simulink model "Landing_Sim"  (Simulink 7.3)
settings: Solver=ode45  StartTime=0.0  StopTime=80  RelTol=1e-3
InitFcn:
  | init
StopFcn:
  | pl
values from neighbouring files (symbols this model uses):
  calfa = cos(alfa0*d2r)    [init.m]
  d2r = pi/180    (= 0.0174532925199)    [init.m]    (also in robust.m)
  ge = 32.174    [init.m]
  r2d = 180/pi    (= 57.2957795131)    [init.m]    (also in robust.m)
  salfa = sin(alfa0*d2r)    [init.m]
  Thet0 = 27.69    [init.m]
  V0 = 24675.1    [init.m]
  x0 = [0 0 -2 -2 0 0 18 0 0 0]'*d2r    [init.m]
undefined symbols (not defined in the file or in its folder): As, Bs, Cs, Ds, KmixM0p4, Kpr, Kq, sigbuilder_block

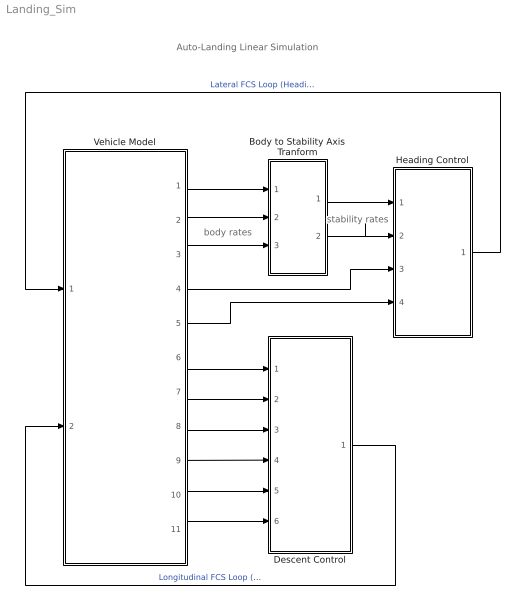
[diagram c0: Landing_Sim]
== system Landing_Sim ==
  note: Auto-Landing Linear Simulation
  note: body rates
  note: stability rates
  Body to Stability Axis Tranform : Subsystem
  Descent Control : Subsystem
  Heading Control : Subsystem
  Vehicle Model : Subsystem
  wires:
  Heading Control/1((dP,dR)) -> Vehicle Model/1("(dP, dR)")  "Lateral FCS Loop (Heading Control)"
  Descent Control/1((dQ  dV)) -> Vehicle Model/2("(dQ, dV)")  "Longitudinal FCS Loop (H, V) control"
  Vehicle Model/3(r) -> Body to Stability Axis Tranform/3(r_b)
  Vehicle Model/2(p) -> Body to Stability Axis Tranform/2(p_b)
  Vehicle Model/1(phi) -> Body to Stability Axis Tranform/1(phi)
  Body to Stability Axis Tranform/1(p_s) -> Heading Control/1(ps)
  Body to Stability Axis Tranform/2(r_s) -> Heading Control/2(rs)
  Vehicle Model/5(Vcr) -> Heading Control/4(Vcr)
  Vehicle Model/4(Ny) -> Heading Control/3(Ny)
  Vehicle Model/6(theta) -> Descent Control/1(theta)
  Vehicle Model/7(q) -> Descent Control/2(q)
  Vehicle Model/8(dH) -> Descent Control/3(dH)
  Vehicle Model/9(dV) -> Descent Control/4(Vel)
  Vehicle Model/10(Nz) -> Descent Control/5(Nz)
  Vehicle Model/11(h-dot) -> Descent Control/6(hdot)

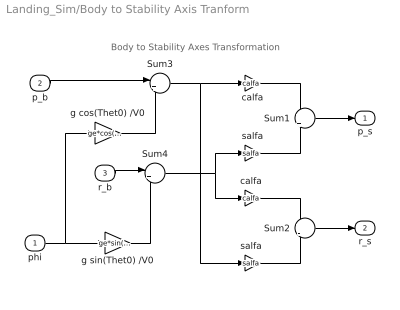
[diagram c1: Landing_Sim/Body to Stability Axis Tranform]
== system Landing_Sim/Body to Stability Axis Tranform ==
  note: Body to Stability Axes Transformation
  phi : Inport  OutDataType=sfix(16)  OutScaling=2^0
  p_b : Inport  Port=2  OutDataType=sfix(16)  OutScaling=2^0
  r_b : Inport  Port=3  OutDataType=sfix(16)  OutScaling=2^0
  Sum1 : Sum  Inputs=+|+  OutDataType=sfix(16)  OutScaling=2^0
  Sum2 : Sum  Inputs=+|-  OutDataType=sfix(16)  OutScaling=2^0
  Sum3 : Sum  Inputs=|++  OutDataType=sfix(16)  OutScaling=2^0
  Sum4 : Sum  Inputs=|+-  OutDataType=sfix(16)  OutScaling=2^0
  calfa : Gain  Gain=calfa  ParameterDataType=sfix(16)  ParameterScaling=2^0  OutDataType=sfix(16)  OutScaling=2^0
  "calfa " : Gain  Gain=calfa  ParameterDataType=sfix(16)  ParameterScaling=2^0  OutDataType=sfix(16)  OutScaling=2^0
  g cos(Thet0) /V0 : Gain  Gain=ge*cos(Thet0*d2r)/V0  ParameterDataType=sfix(16)  ParameterScaling=2^0  OutDataType=sfix(16)  OutScaling=2^0
  g sin(Thet0) /V0 : Gain  Gain=ge*sin(Thet0*d2r)/V0  ParameterDataType=sfix(16)  ParameterScaling=2^0  OutDataType=sfix(16)  OutScaling=2^0
  salfa : Gain  Gain=salfa  ParameterDataType=sfix(16)  ParameterScaling=2^0  OutDataType=sfix(16)  OutScaling=2^0
  "salfa " : Gain  Gain=salfa  ParameterDataType=sfix(16)  ParameterScaling=2^0  OutDataType=sfix(16)  OutScaling=2^0
  p_s : Outport  OutDataType=sfix(16)  OutScaling=2^0
  r_s : Outport  Port=2  OutDataType=sfix(16)  OutScaling=2^0
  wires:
  Sum1/1 -> p_s/1
  Sum2/1 -> r_s/1
  p_b/1 -> Sum3/1
  r_b/1 -> Sum4/1
  g cos(Thet0) /V0/1 -> Sum3/2
  g sin(Thet0) /V0/1 -> Sum4/2
  phi/1 -> g cos(Thet0) /V0/1, g sin(Thet0) /V0/1
  Sum4/1 -> "calfa "/1, salfa/1
  Sum3/1 -> "salfa "/1, calfa/1
  calfa/1 -> Sum1/1
  salfa/1 -> Sum1/2
  "calfa "/1 -> Sum2/1
  "salfa "/1 -> Sum2/2

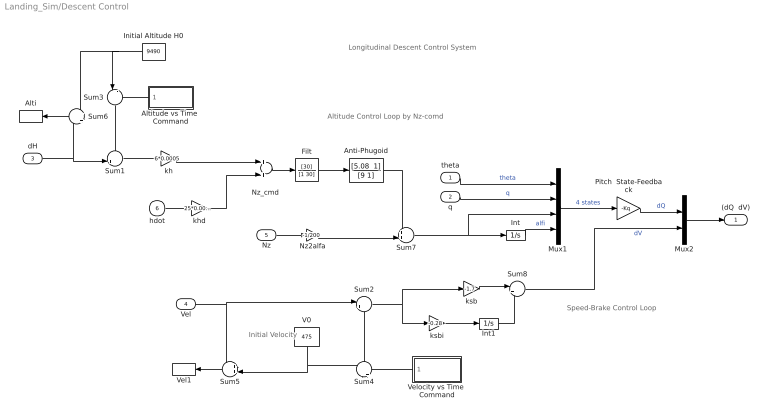
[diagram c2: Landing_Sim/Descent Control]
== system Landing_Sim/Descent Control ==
  note: Longitudinal Descent Control System
  note: Initial Velocity
  note: Altitude Control Loop by Nz-comd
  note: Speed-Brake Control Loop
  theta : Inport
  q : Inport  Port=2
  dH : Inport  Port=3
  Vel : Inport  Port=4
  Nz : Inport  Port=5
  hdot : Inport  Port=6  OutDataType=sfix(16)  OutScaling=2^0
  Alti : ToWorkspace  VariableName=Alti  SampleTime=-1  SaveFormat=Array
  Altitude vs Time  Command : Subsystem  Tag=STV Subsys  LoadFcn=sigbuilder_block('load');  StartFcn=sigbuilder_block('start');  StopFcn=sigbuilder_block('stop');  ClipboardFcn=sigbuilder_block('clipboard');
  Anti-Phugoid : TransferFcn  Numerator="[5.08  1]"  Denominator=[9 1]
  Filt : TransferFcn  Numerator=[30]  Denominator=[1 30]
  Initial Altitude H0 : Constant  Value=9490  OutDataType=fixdt(1, 16)  OutScaling=2^0
  Int : Integrator
  Int1 : Integrator
  Mux1 : Mux
  Mux2 : Mux  Inputs=2
  Nz2alfa : Gain  Gain=-1/200  ParameterDataType=sfix(16)  ParameterScaling=2^0  OutDataType=sfix(16)  OutScaling=2^0
  "Nz_cmd " : Sum  OutDataType=sfix(16)  OutScaling=2^0
  Pitch  State-Feedback : Gain  Gain=-Kq  Multiplication=Matrix(K*u)  ParameterDataType=sfix(16)  ParameterScaling=2^0  OutDataType=sfix(16)  OutScaling=2^0
  Sum1 : Sum  Inputs=-+|  OutDataType=sfix(16)  OutScaling=2^0
  Sum2 : Sum  Inputs=|+-  OutDataType=sfix(16)  OutScaling=2^0
  Sum3 : Sum  Inputs=|-+  OutDataType=sfix(16)  OutScaling=2^0
  Sum4 : Sum  Inputs=-|+  OutDataType=sfix(16)  OutScaling=2^0
  Sum5 : Sum  Inputs=++|  OutDataType=sfix(16)  OutScaling=2^0
  Sum6 : Sum  Inputs=+|+  OutDataType=sfix(16)  OutScaling=2^0
  Sum7 : Sum  Inputs=++|  OutDataType=sfix(16)  OutScaling=2^0
  Sum8 : Sum  Inputs=|++  OutDataType=sfix(16)  OutScaling=2^0
  V0 : Constant  Value=475  OutDataType=fixdt(1, 16)  OutScaling=2^0
  Vel1 : ToWorkspace  VariableName=Vel  SampleTime=-1  SaveFormat=Array
  Velocity vs Time  Command : Subsystem  Tag=STV Subsys  LoadFcn=sigbuilder_block('load');  StartFcn=sigbuilder_block('start');  StopFcn=sigbuilder_block('stop');  ClipboardFcn=sigbuilder_block('clipboard');
  kh : Gain  Gain=6*0.0005  ParameterDataType=sfix(16)  ParameterScaling=2^0  OutDataType=sfix(16)  OutScaling=2^0
  khd : Gain  Gain=25*0.0005  ParameterDataType=sfix(16)  ParameterScaling=2^0  OutDataType=sfix(16)  OutScaling=2^0
  ksb : Gain  Gain=-1.7  ParameterDataType=sfix(16)  ParameterScaling=2^0  OutDataType=sfix(16)  OutScaling=2^0
  ksbi : Gain  Gain=-0.28  ParameterDataType=sfix(16)  ParameterScaling=2^0  OutDataType=sfix(16)  OutScaling=2^0
  (dQ  dV) : Outport
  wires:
  dH/1 -> Sum1/2, Sum6/2
  Altitude vs Time  Command/1(altit) -> Sum3/2
  Initial Altitude H0/1 -> Sum3/1, Sum6/1
  Sum6/1 -> Alti/1
  Vel/1 -> Sum2/1, Sum5/1
  Sum2/1 -> ksb/1, ksbi/1
  Sum5/1 -> Vel1/1
  Velocity vs Time  Command/1(veloc) -> Sum4/2
  theta/1 -> Mux1/1  "theta"
  q/1 -> Mux1/2  "q"
  Int/1 -> Mux1/4  "alfi"
  Sum7/1 -> Int/1, Mux1/3
  Mux1/1 -> Pitch  State-Feedback/1  "4 states"
  Pitch  State-Feedback/1 -> Mux2/1  "dQ"
  "Nz_cmd "/1 -> Filt/1
  hdot/1 -> khd/1
  khd/1 -> "Nz_cmd "/2
  Sum1/1 -> kh/1
  ksb/1 -> Sum8/1
  ksbi/1 -> Int1/1
  Mux2/1 -> (dQ  dV)/1
  Nz/1 -> Nz2alfa/1
  Int1/1 -> Sum8/2
  Sum8/1 -> Mux2/2  "dV"
  Nz2alfa/1 -> Sum7/2
  V0/1 -> Sum5/2, Sum4/1
  Sum4/1 -> Sum2/2
  Sum3/1 -> Sum1/1
  kh/1 -> "Nz_cmd "/1
  Filt/1 -> Anti-Phugoid/1
  Anti-Phugoid/1 -> Sum7/1

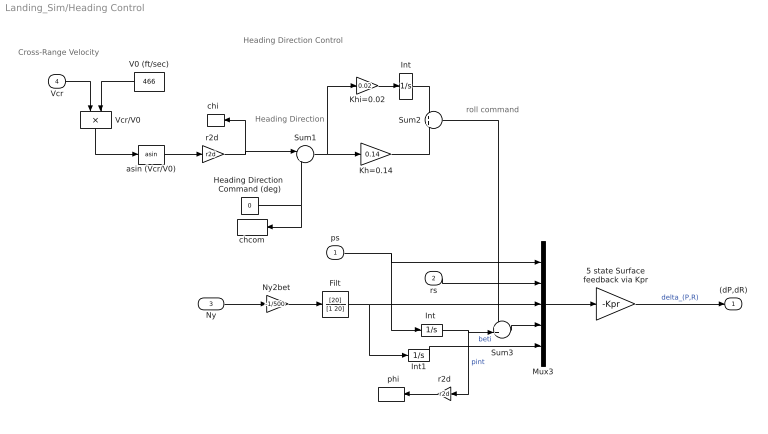
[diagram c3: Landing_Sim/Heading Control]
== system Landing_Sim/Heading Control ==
  note: Heading Direction Control
  note: roll command
  note: Heading Direction
  note: Cross-Range Velocity
  ps : Inport  OutDataType=sfix(16)  OutScaling=2^0
  rs : Inport  Port=2  OutDataType=sfix(16)  OutScaling=2^0
  Ny : Inport  Port=3
  Vcr : Inport  Port=4  OutDataType=sfix(16)  OutScaling=2^0
  "  phi" : ToWorkspace  VariableName=phist  SampleTime=-1  SaveFormat=Array
  5 state Surface feedback via Kpr : Gain  Gain=-Kpr  Multiplication=Matrix(K*u)  ParameterDataType=sfix(16)  ParameterScaling=2^0  OutDataType=sfix(16)  OutScaling=2^0
  Filt : TransferFcn  Numerator=[20]  Denominator=[1 20]
  Heading Direction  Command (deg) : Constant  Value=0  OutDataType=sfix(16)  OutScaling=2^0
  Int : Integrator
  "Int " : Integrator
  Int1 : Integrator
  Kh=0.14 : Gain  Gain=0.14  ParameterDataType=sfix(16)  ParameterScaling=2^0  OutDataType=sfix(16)  OutScaling=2^0
  Khi=0.02 : Gain  Gain=0.02  ParameterDataType=sfix(16)  ParameterScaling=2^0  OutDataType=sfix(16)  OutScaling=2^0
  Mux3 : Mux  Inputs=5
  "Ny2bet " : Gain  Gain=-1/500  ParameterDataType=sfix(16)  ParameterScaling=2^0  OutDataType=sfix(16)  OutScaling=2^0
  Sum1 : Sum  Inputs=|+-  OutDataType=sfix(16)  OutScaling=2^0
  Sum2 : Sum  OutDataType=sfix(16)  OutScaling=2^0
  Sum3 : Sum  Inputs=++|  OutDataType=sfix(16)  OutScaling=2^0
  V0 (ft/sec) : Constant  Value=466  OutDataType=sfix(16)  OutScaling=2^0
  Vcr/V0 : Product  Inputs=*/  OutDataType=sfix(16)  OutScaling=2^0
  asin (Vcr/V0) : Trigonometry  Operator=asin
  chcom : ToWorkspace  VariableName=chicm  SampleTime=-1  SaveFormat=Array
  "chi  " : ToWorkspace  VariableName=chi  SampleTime=-1  SaveFormat=Array
  r2d : Gain  Gain=r2d  ParameterDataType=sfix(16)  ParameterScaling=2^0  OutDataType=sfix(16)  OutScaling=2^0
  "r2d " : Gain  Gain=r2d  ParameterDataType=sfix(16)  ParameterScaling=2^0  OutDataType=sfix(16)  OutScaling=2^0
  (dP,dR) : Outport  OutDataType=sfix(16)  OutScaling=2^0
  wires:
  Heading Direction  Command (deg)/1 -> Sum1/2, chcom/1
  Vcr/1 -> Vcr/V0/1
  Sum1/1 -> Kh=0.14/1, Khi=0.02/1
  Sum2/1 -> Sum3/1
  Int/1 -> Sum2/1
  Kh=0.14/1 -> Sum2/2
  Khi=0.02/1 -> Int/1
  "r2d "/1 -> Sum1/1, "chi  "/1
  Vcr/V0/1 -> asin (Vcr/V0)/1
  asin (Vcr/V0)/1 -> "r2d "/1
  V0 (ft/sec)/1 -> Vcr/V0/2
  Mux3/1 -> 5 state Surface feedback via Kpr/1
  5 state Surface feedback via Kpr/1 -> (dP,dR)/1  "delta_(P,R)"
  r2d/1 -> "  phi"/1
  rs/1 -> Mux3/2
  ps/1 -> "Int "/1, Mux3/1
  Int1/1 -> Mux3/5  "beti"
  Sum3/1 -> Mux3/4
  "Int "/1 -> r2d/1, Sum3/2  "pint"
  "Ny2bet "/1 -> Filt/1
  Ny/1 -> "Ny2bet "/1
  Filt/1 -> Int1/1, Mux3/3

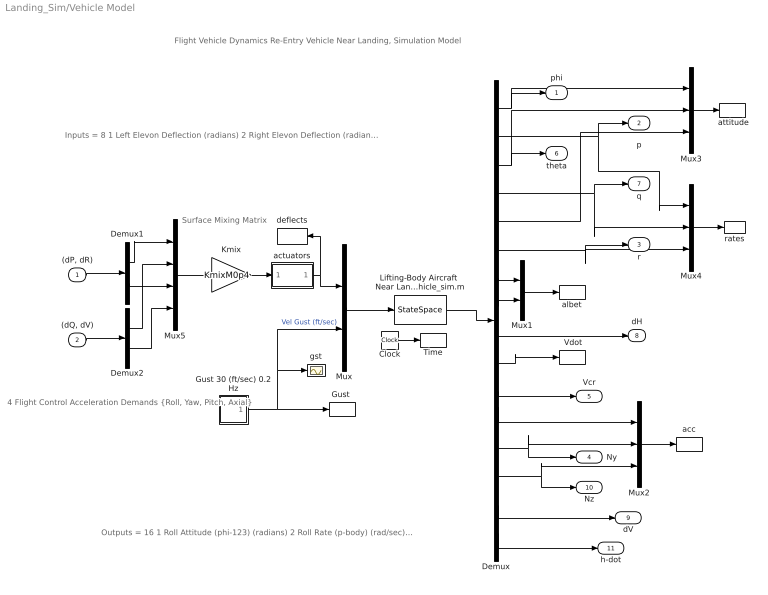
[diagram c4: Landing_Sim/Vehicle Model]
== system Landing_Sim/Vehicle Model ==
  note: Flight Vehicle Dynamics Re-Entry Vehicle Near Landing, Simulation Model
  note: Surface Mixing Matrix
  note: Outputs = 16 1 Roll Attitude (phi-123) (radians) 2 Roll Rate (p-body) (rad/sec) 3 Pitch Attitude (thet-123) (radians) 4 Pitch Rate (q-body) (rad/sec) 5 Yaw Attitude (psi-123) (radians) 6 Yaw Rate (r-body) (rad/sec) 7 Angle of attack, alfa, (radians) 8 Angle of sideslip, beta, (radian) 9 Change in Altitude, delta-h, (feet) 10 Forward Acceleration (V-dot) (ft/sec) 11 Cross Range Velocity (Vcr) (ft/sec) 12 Accelerom # 1, (along X), (ft/sec^2) Translat. Acceler 13 Accelerom # 2, (along Y), (ft/sec^2) Translat. Acceler 14 Accelerom # 3, (along Z), (ft/sec^2) Translat. Acceler 15 Change in Velocity (delta-V) (ft/sec) 16 Altitude Rate (h-dot) (ft/sec)
  note: 4 Flight Control Acceleration Demands {Roll, Yaw, Pitch, Axial}
  note: Inputs = 8 1 Left Elevon Deflection (radians) 2 Right Elevon Deflection (radians) 3 Vertical Rudder Deflection (radians) 4 Upper Left Body-Flap Deflection (radians) 5 Upper Right Body-Flap Deflection (radians) 6 Lower Left Body-Flap Deflection (radians) 7 Lower Right Body-Flap Deflection (radians) 8 Wind Gust Azim & Elev Angles =(45, 90) (deg)
  "(dP, dR)" : Inport  OutDataType=sfix(16)  OutScaling=2^0
  "(dQ, dV)" : Inport  Port=2  OutDataType=sfix(16)  OutScaling=2^0
  " Vdot" : ToWorkspace  VariableName=Vdot  SampleTime=-1  SaveFormat=Array
  " attitude" : ToWorkspace  VariableName=atti  SampleTime=-1  SaveFormat=Array
  Clock : Clock
  Demux : Demux  Outputs=16
  Demux1 : Demux  Outputs=2
  Demux2 : Demux  Outputs=2
  Gust 30 (ft/sec) 0.2 Hz : Subsystem
  "Gust " : ToWorkspace  VariableName=Gust  SampleTime=-1  SaveFormat=Array
  Kmix : Gain  Gain=KmixM0p4  Multiplication=Matrix(K*u)  ParameterDataType=sfix(16)  ParameterScaling=2^0  OutDataType=sfix(16)  OutScaling=2^0
  "Lifting-Body Aircraft  Near Landing,  Simulation Model  from file vehicle_sim.m" : StateSpace  A=As  B=Bs  C=Cs  D=Ds  X0=x0
  Mux : Mux  Inputs=[7,1]
  Mux1 : Mux  Inputs=2
  Mux2 : Mux  Inputs=3
  Mux3 : Mux  Inputs=3
  Mux4 : Mux  Inputs=3
  Mux5 : Mux
  Time : ToWorkspace  VariableName=time  SampleTime=-1  SaveFormat=Array
  acc : ToWorkspace  VariableName=acc  SampleTime=-1  SaveFormat=Array
  actuators : Subsystem
  albet : ToWorkspace  VariableName=albet  SampleTime=-1  SaveFormat=Array
  deflects : ToWorkspace  VariableName=Surf  SampleTime=-1  SaveFormat=Array
  gst : Scope
  rates : ToWorkspace  VariableName=pqr  SampleTime=-1  SaveFormat=Array
  phi : Outport  OutDataType=sfix(16)  OutScaling=2^0
  p : Outport  Port=2  OutDataType=sfix(16)  OutScaling=2^0
  r : Outport  Port=3  OutDataType=sfix(16)  OutScaling=2^0
  Ny : Outport  Port=4  OutDataType=sfix(16)  OutScaling=2^0
  Vcr : Outport  Port=5  OutDataType=sfix(16)  OutScaling=2^0
  theta : Outport  Port=6  OutDataType=sfix(16)  OutScaling=2^0
  q : Outport  Port=7  OutDataType=sfix(16)  OutScaling=2^0
  dH : Outport  Port=8  OutDataType=sfix(16)  OutScaling=2^0
  dV : Outport  Port=9  OutDataType=sfix(16)  OutScaling=2^0
  Nz : Outport  Port=10  OutDataType=sfix(16)  OutScaling=2^0
  h-dot : Outport  Port=11  OutDataType=sfix(16)  OutScaling=2^0
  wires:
  Mux/1 -> "Lifting-Body Aircraft  Near Landing,  Simulation Model  from file vehicle_sim.m"/1
  Gust 30 (ft/sec) 0.2 Hz/1(Gust) -> "Gust "/1, gst/1, Mux/2  "Vel Gust (ft/sec)"
  Clock/1 -> Time/1
  "Lifting-Body Aircraft  Near Landing,  Simulation Model  from file vehicle_sim.m"/1 -> Demux/1
  Kmix/1 -> actuators/1(In)
  actuators/1(out) -> Mux/1, deflects/1
  Demux/1 -> phi/1, Mux3/1
  Demux/3 -> theta/1, Mux3/2
  Demux/5 -> Mux3/3
  Demux/2 -> p/1, Mux4/1
  Demux/4 -> q/1, Mux4/2
  Demux/6 -> r/1, Mux4/3
  Demux/8 -> Mux1/2
  Demux/7 -> Mux1/1
  Mux1/1 -> albet/1
  Demux/9 -> dH/1
  Demux/15 -> dV/1
  Demux/12 -> Mux2/1
  Demux/13 -> Mux2/2, Ny/1
  Demux/14 -> Mux2/3, Nz/1
  Mux2/1 -> acc/1
  Demux/11 -> Vcr/1
  Mux3/1 -> " attitude"/1
  Mux4/1 -> rates/1
  Demux/10 -> " Vdot"/1
  Mux5/1 -> Kmix/1
  Demux1/1 -> Mux5/1
  Demux1/2 -> Mux5/3
  Demux2/1 -> Mux5/2
  Demux2/2 -> Mux5/4
  "(dP, dR)"/1 -> Demux1/1
  "(dQ, dV)"/1 -> Demux2/1
  Demux/16 -> h-dot/1

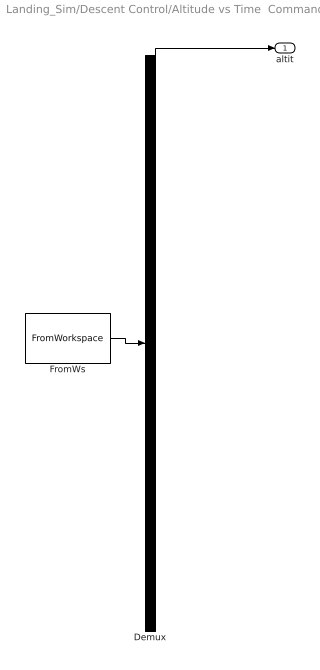
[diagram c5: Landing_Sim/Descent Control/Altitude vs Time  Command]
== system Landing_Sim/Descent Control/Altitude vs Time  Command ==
  Demux : Demux  Tag=STV Demux  Outputs=1
  FromWs : FromWorkspace  Tag=STV FromWs  VariableName=tuvar  SampleTime=0  SigBuilderData=DataTag0  VnvData=DataTag1
  altit : Outport  Tag=STV Outport
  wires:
  FromWs/1 -> Demux/1
  Demux/1 -> altit/1

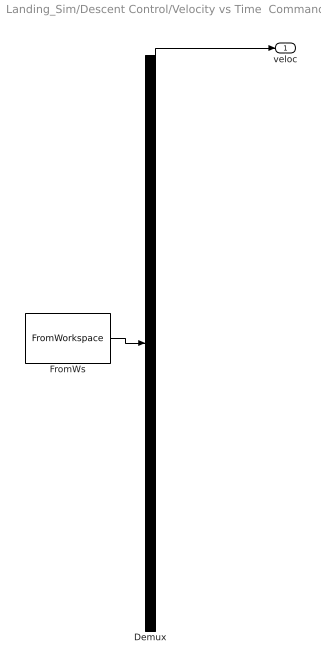
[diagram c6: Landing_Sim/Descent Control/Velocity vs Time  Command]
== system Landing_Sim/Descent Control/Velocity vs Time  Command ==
  Demux : Demux  Tag=STV Demux  Outputs=1
  FromWs : FromWorkspace  Tag=STV FromWs  VariableName=tuvar  SampleTime=0  SigBuilderData=DataTag2  VnvData=DataTag3
  veloc : Outport  Tag=STV Outport
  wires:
  FromWs/1 -> Demux/1
  Demux/1 -> veloc/1

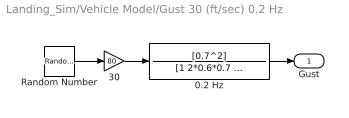
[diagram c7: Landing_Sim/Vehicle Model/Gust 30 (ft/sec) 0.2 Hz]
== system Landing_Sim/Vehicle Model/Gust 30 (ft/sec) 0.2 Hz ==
  0.2 Hz : TransferFcn  Numerator=[0.7^2]  Denominator="[1 2*0.6*0.7  0.7^2]"
  30 : Gain  Gain=80  ParameterDataType=sfix(16)  ParameterScaling=2^0  OutDataType=sfix(16)  OutScaling=2^0
  Random Number : RandomNumber  SampleTime=0
  Gust : Outport  OutDataType=sfix(16)  OutScaling=2^0
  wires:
  30/1 -> 0.2 Hz/1
  Random Number/1 -> 30/1
  0.2 Hz/1 -> Gust/1

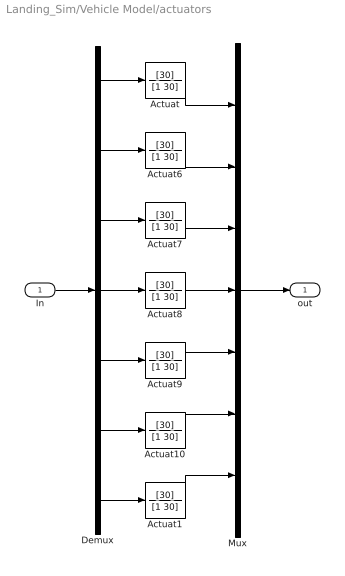
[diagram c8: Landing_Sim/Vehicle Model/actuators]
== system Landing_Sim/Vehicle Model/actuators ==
  In : Inport
  Actuat{,1,6..10} (7 alike) : TransferFcn  Numerator=[30]  Denominator=[1 30]
  Demux : Demux  Outputs=7
  Mux : Mux  Inputs=7
  out : Outport
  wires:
  Actuat10/1 -> Mux/6
  Actuat9/1 -> Mux/5
  Actuat8/1 -> Mux/4
  Actuat7/1 -> Mux/3
  Actuat6/1 -> Mux/2
  Actuat/1 -> Mux/1
  Demux/6 -> Actuat10/1
  Demux/5 -> Actuat9/1
  Demux/4 -> Actuat8/1
  Demux/3 -> Actuat7/1
  Demux/2 -> Actuat6/1
  Demux/1 -> Actuat/1
  Demux/7 -> Actuat1/1
  Actuat1/1 -> Mux/7
  Mux/1 -> out/1
  In/1 -> Demux/1
